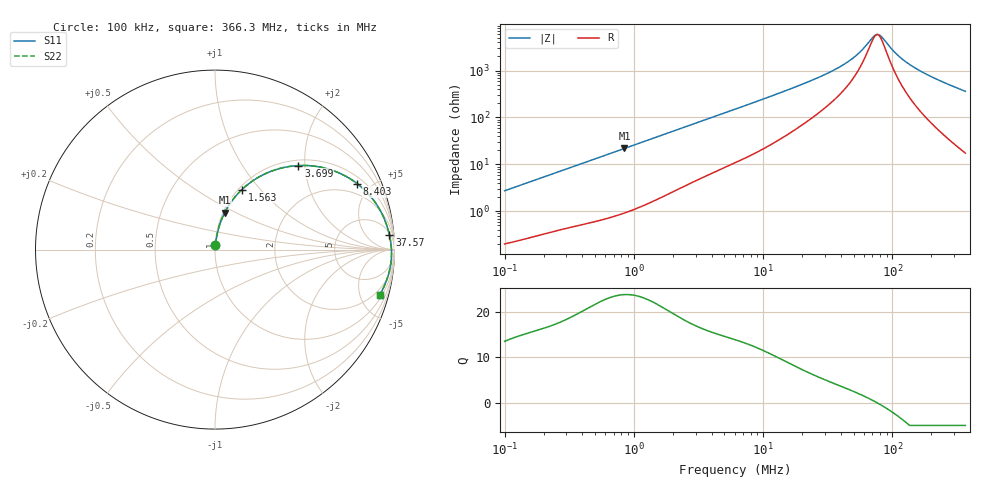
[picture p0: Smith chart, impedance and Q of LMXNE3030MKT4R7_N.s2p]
! LMXNE3030MKT4R7_N  S-PARAMETER MODEL  ( General Type )
! Model Generated by TAIYO YUDEN Corporation (http://www.ty-top.com)
! Version 1.0
! TAIYO YUDEN Control No. 191023NI43SB-FBB
! Copyright(c) 2019 TAIYO YUDEN CO.,LTD. All Rights Reserved.
! Product Description (link to TY-COMPAS)
! https://ds.yuden.co.jp/TYCOMPAS/or/detail?pn=LMXNE3030MKT4R7MN&u=M
! Products Name : Inductors
! Characteristics :
!  Inductance : 4.7 uH , SRF(min) : 50 MHz , DC Resistance(max) : 0.156 Ohm
!  Rated Current : Saturation :1000 mA , Temp Rise : 1060 mA
!  Case Size : 3.0 x 3.0 / 0.118 x 0.118 [mm/inch] , Thickness : 1.2 / 0.047 [mm/inch]
!  (Conditions: Temperature = 25 degC , DC Bias Current/Voltage = 0A / 0V)
! External Node Assignments :
!  1  o---GGG---o  2
! GND o---------o GND
! Frequency Range : 0.1MHz  -  366.261039MHz  [ 402 STEP ]
# MHz S RI R 50
! Freq[MHz].  S11 Real  S11 Imag  S21 Real  S21 Imag  S12 Real  S12 Imag  S22 Real  S22 Imag
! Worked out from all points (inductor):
!   401 points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, 100 kHz to 366.3 MHz, reference 50 ohm
!   read as one part in series: L = 4.33 uH near 104.2 kHz
!   highest Q = 23.8 at 844.5 kHz (marker M1), where L = 4.13 uH
!   self-resonance near 75.98 MHz
!   S11 on the Smith chart (normalised r, x): 100 kHz: 1.00, +0.05; 1.563 MHz: 1.04, +0.80; 3.699 MHz: 1.12, +1.85; 8.403 MHz: 1.33, +4.13; 37.57 MHz: 7, +22; 366.3 MHz: 1.35, -7.20
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0.1  0.00276 0.0272  0.9972 -0.0272  0.9972 -0.0272  0.00276 0.0272
0.395307  0.0157 0.1018  0.9843 -0.1018  0.9843 -0.1018  0.0157 0.1018
0.844473  0.0537 0.2054  0.9463 -0.2054  0.9463 -0.2054  0.0537 0.2054
1.562679  0.1502 0.3347  0.8498 -0.3347  0.8498 -0.3347  0.1502 0.3347
2.307544  0.2676 0.4167  0.7324 -0.4167  0.7324 -0.4167  0.2676 0.4167
3.69886  0.4652 0.4683  0.5348 -0.4683  0.5348 -0.4683  0.4652 0.4683
6.177387  0.6881 0.4285  0.3119 -0.4285  0.3119 -0.4285  0.6881 0.4285
8.403244  0.7929 0.367  0.2071 -0.367  0.2071 -0.367  0.7929 0.367
13.46992  0.8958 0.2584  0.1042 -0.2584  0.1042 -0.2584  0.8958 0.2584
23.92381  0.9527 0.147  0.0473 -0.147  0.0473 -0.147  0.9527 0.147
37.56979  0.9717 0.0819  0.0283 -0.0819  0.0283 -0.0819  0.9717 0.0819
45.1881  0.9763 0.0591  0.0237 -0.0591  0.0237 -0.0591  0.9763 0.0591
52.16635  0.979 0.0424  0.021 -0.0424  0.021 -0.0424  0.979 0.0424
69.52214  0.9826 0.00998  0.0174 -0.00998  0.0174 -0.00998  0.9826 0.00998
73.93525  0.9831 0.00307  0.0169 -0.00307  0.0169 -0.00307  0.9831 0.00307
77.03188  0.9833 -0.00156  0.0167 0.00156  0.0167 0.00156  0.9833 -0.00156
80.2582  0.9835 -0.00621  0.0165 0.00621  0.0165 0.00621  0.9835 -0.00621
94.57258  0.9837 -0.0252  0.0163 0.0252  0.0163 0.0252  0.9837 -0.0252
118.514  0.9824 -0.0527  0.0176 0.0527  0.0176 0.0527  0.9824 -0.0527
154.7365  0.9779 -0.0888  0.0221 0.0888  0.0221 0.0888  0.9779 -0.0888
228.4929  0.9625 -0.1521  0.0375 0.1521  0.0375 0.1521  0.9625 -0.1521
366.261  0.9182 -0.251  0.0818 0.251  0.0818 0.251  0.9182 -0.251
